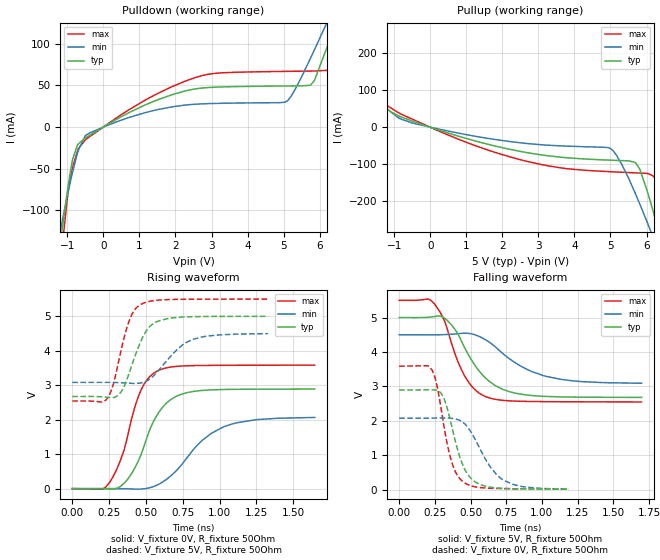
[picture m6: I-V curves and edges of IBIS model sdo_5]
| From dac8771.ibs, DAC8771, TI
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|   sdo_5 Model
[Model]   sdo_5
Model_type   Output
Polarity   Non-Inverting
Vmeas = 2.5
Vref = 0
Cref = 2pF
Rref = 70
|   typ   min   max
|   (nom PVT)   (fast PVT)   (slow PVT)
C_comp   2.914e-12   2.914e-12   2.914e-12
| Where nom  PVT is Nominal Process, 5V, 27C
|   Fast PVT is Strong Process,  5.5V, -40C
|   Slow PVT is Weak Process,   4.5V, 150C
[Voltage Range]   5   4.5   5.5
|Junction Temperature
[Temperature Range]   27   150   -40
[Pullup Reference]   5   4.5   5.5
[Pulldown Reference]   0   0   0
[Power Clamp Reference]   5   4.5   5.5
[GND Clamp Reference]   0   0   0
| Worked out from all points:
|   slope of the pulldown table from 0 to 0.75 V, typ, clamps not added: 41.4 ohm
|   slope of the pullup table from 0 to 0.75 V, typ, clamps not added: 32.1 ohm
|   falling waveform, V_fixture 5V, R_fixture 50Ohm: 20-80 % time 222ps typ, 316ps min, 168ps max; typ from 5 V to 2.68 V
|   rising waveform, V_fixture 0V, R_fixture 50Ohm: 20-80 % time 182ps typ, 285ps min, 150ps max; typ from 0 V to 2.88 V
|   rising waveform, V_fixture 5V, R_fixture 50Ohm: 20-80 % time 128ps typ, 191ps min, 105ps max; typ from 2.67 V to 5 V
|   falling waveform, V_fixture 0V, R_fixture 50Ohm: 20-80 % time 120ps typ, 180ps min, 102ps max; typ from 2.89 V to 0.014 V
[Pulldown]
|   Voltage   I(typ)   I(min)   I(max)
-5V       -1.575A    -1.155A    -1.985A
-1.135V   -119.8mA   -111.2mA   -140.8mA
-896mV    -48.48mA   -61.77mA   -55.74mA
-693.5mV  -20.09mA   -27.46mA   -25.87mA
-374mV    -9.624mA   -6.839mA   -11.26mA
1.506V    32.84mA    21.03mA    40.42mA
2.914V    47.55mA    28.22mA    63.51mA
5.04V     49.39mA    29.98mA    66.92mA
5.745V    50.27mA    82.65mA    67.29mA
6.324V    109.6mA    137mA      68.46mA
7.21V     222.6mA    222.7mA    196mA
10V       612.2mA    513.5mA    696.7mA
[Pullup]
|   Voltage   I(typ)   I(min)   I(max)
-5V       528.8mA    411.8mA    677.1mA
-2.415V   196.7mA    163mA      243.2mA
-1.31V    60.42mA    59.69mA    67.74mA
-500mV    16.42mA    11.2mA     21.64mA
2.5V      -65.74mA   -42.42mA   -88.14mA
4.999V    -89.45mA   -57.92mA   -120.6mA
5.695V    -96mA      -180.9mA   -123.8mA
6.044V    -181.2mA   -263.8mA   -125.7mA
6.181V    -226.9mA   -298mA     -132mA
6.313V    -272.6mA   -331.4mA   -148.6mA
6.77V     -438.9mA   -451mA     -327.9mA
10V       -1.674A    -1.363A    -1.883A
[Ramp]
R_load = 50
|   typ   min   max
dV/dt_r   1.73587/1.82729e-10   1.24566/2.85416e-10   2.15197/1.50665e-10
dV/dt_f   1.39807/2.24531e-10   0.852693/3.17683e-10   1.77701/1.68166e-10
[Falling Waveform]
V_fixture = 5V
V_fixture_min = 4.5V
V_fixture_max = 5.5V
R_fixture = 50Ohm
|   Time   V(typ)   V(min)   V(max)
0s        5V         4.5V       5.5V
200.6ps   5.007V     4.499V     5.537V
244.8ps   5.028V     4.499V     5.409V
337.8ps   4.911V     4.508V     4.657V
404.6ps   4.572V     4.528V     3.796V
458.4ps   4.127V     4.545V     3.309V
607.9ps   3.232V     4.346V     2.7V
770.4ps   2.85V      3.809V     2.581V
1.021ns   2.709V     3.301V     2.557V
1.698ns   2.68V      3.091V     2.547V
[Rising Waveform]
V_fixture = 0V
V_fixture_min = 0V
V_fixture_max = 0V
R_fixture = 50Ohm
|   Time   V(typ)   V(min)   V(max)
0s        3.128nV    19.47nV    3.02nV
202.8ps   -3.105mV   1.039mV    -14.43mV
252.5ps   -14.88mV   1.272mV    172.1mV
349.4ps   143.6mV    -3.021mV   1.09V
465.2ps   966.1mV    -12.51mV   2.841V
583.3ps   2.183V     117.7mV    3.421V
734.1ps   2.725V     647mV      3.552V
876.7ps   2.844V     1.375V     3.569V
1.021ns   2.873V     1.778V     3.574V
1.647ns   2.885V     2.063V     3.58V
[Rising Waveform]
V_fixture = 5V
V_fixture_min = 4.5V
V_fixture_max = 5.5V
R_fixture = 50Ohm
|   Time   V(typ)   V(min)   V(max)
0s        2.67V      3.079V     2.538V
240.8ps   2.647V     3.08V      2.634V
279.3ps   2.64V      3.077V     3.036V
337.8ps   2.846V     3.068V     4.129V
395.3ps   3.461V     3.054V     4.96V
469.2ps   4.305V     3.066V     5.347V
572.1ps   4.834V     3.36V      5.46V
716.1ps   4.964V     4.048V     5.487V
811.3ps   4.983V     4.317V     5.49V
1.33ns    4.995V     4.493V     5.495V
[Falling Waveform]
V_fixture = 0V
V_fixture_min = 0V
V_fixture_max = 0V
R_fixture = 50Ohm
|   Time   V(typ)   V(min)   V(max)
0s        2.893V     2.076V     3.587V
230.2ps   2.901V     2.078V     3.474V
262.9ps   2.887V     2.081V     3.066V
311.3ps   2.675V     2.083V     1.91V
370.1ps   1.811V     2.07V      774.8mV
458.4ps   599.9mV    1.917V     197.4mV
545.5ps   194.4mV    1.356V     73.04mV
639.4ps   71.51mV    654.4mV    39.83mV
728.9ps   36.88mV    281.7mV    30.1mV
1.189ns   14.46mV    16.4mV     17.77mV
